{attribute 'no_assign'}
FUNCTION_BLOCK FB_LN_IED_MUnn_LPHD1 EXTENDS FB_AcsiCommonLogicalNodeClass
VAR_INPUT
	PhyNam: FB_DO_IED_MUnn_LPHD1_PhyNam := (sClass:='DPL', bLinkResult:=THIS^.AddDataToContainer(ipData:=PhyNam));
	PhyHealth: FB_DO_IED_MUnn_LPHD1_PhyHealth := (sClass:='ENS', bLinkResult:=THIS^.AddDataToContainer(ipData:=PhyHealth));
	Proxy: FB_DO_IED_MUnn_LPHD1_Proxy := (sClass:='SPS', bLinkResult:=THIS^.AddDataToContainer(ipData:=Proxy));
END_VAR
VAR
END_VAR

END_FUNCTION_BLOCK
